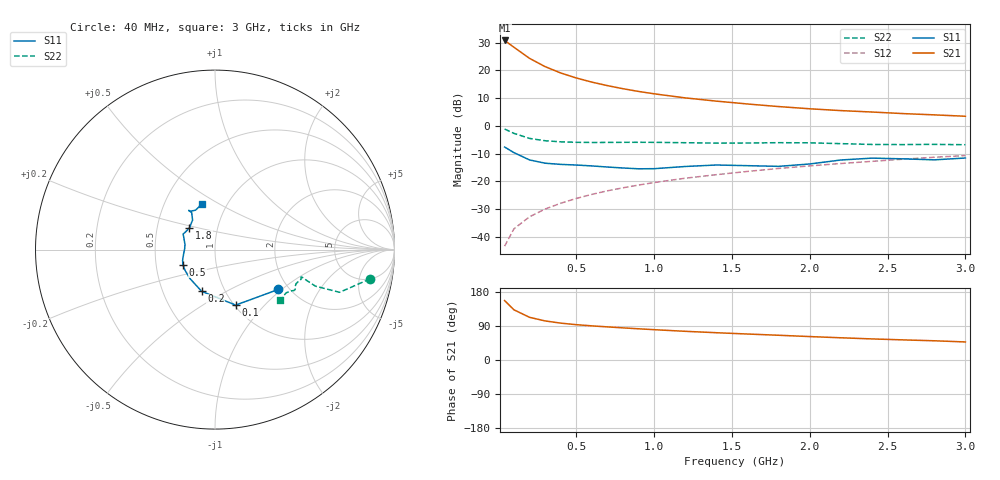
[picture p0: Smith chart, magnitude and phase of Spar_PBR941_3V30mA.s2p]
! Filename:  PBR941H.S2P  Version:  3.0
! NXP part #:  PBR941  Date: July 1998
! Bias condition:  Vce=3V, Ic=30mA
#  MHz  S  MA  R 50
! Freq  S11  S21  S12  S22
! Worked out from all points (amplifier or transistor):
!   21 points, 40 MHz to 3 GHz, reference 50 ohm
!   highest |S21| = 30.8 dB at 40 MHz (marker M1)
!   |S21| within 3 dB of that: start of sweep to 114 MHz
!   unconditionally stable (mu >= 1): 306.6 MHz to 2.554 GHz
!   at 300 MHz: K = 1.00, MSG = 25.6 dB, |S12| = -29.9 dB
!   at 1 GHz: K = 1.10, MAG = 14.1 dB, |S12| = -20.4 dB
!   at 3 GHz: K = 0.99, MSG = 7.1 dB, |S12| = -10.7 dB
!   S11 on the Smith chart (normalised r, x): 40 MHz: 1.76, -0.95; 100 MHz: 1.01, -0.70; 200 MHz: 0.78, -0.38; 500 MHz: 0.69, -0.12; 1.8 GHz: 0.73, +0.18; 3 GHz: 0.77, +0.42
40  0.4167 -32.2  34.49 156.9  0.006845 77.8  0.8788 -10.7
100  0.33 -69.6  26.04 132.4  0.01406 73.2  0.734 -18.9
200  0.244 -107.8  16.44 112.6  0.02313 72.5  0.5951 -20.0
300  0.2131 -131.2  11.67 103.1  0.03187 75.3  0.5406 -18.6
400  0.2029 -145.5  8.971 97.3  0.04049 77.4  0.5168 -17.8
500  0.1976 -155.0  7.289 93.2  0.04941 78.7  0.5065 -17.6
600  0.1903 -161.5  6.14 90.1  0.05851 79.7  0.5032 -17.7
700  0.182 -167.3  5.307 87.4  0.0678 80.7  0.504 -18.0
800  0.1747 -174.0  4.671 84.8  0.07682 80.9  0.5061 -18.4
900  0.169 178.2  4.172 82.4  0.0861 81.0  0.5068 -18.8
1000  0.1698 170.2  3.782 80.0  0.09553 81.0  0.5058 -19.3
1200  0.1859 159.2  3.192 75.7  0.1144 80.7  0.4981 -20.6
1400  0.1978 154.0  2.791 72.0  0.1324 80.3  0.49 -22.8
1600  0.1924 150.1  2.48 68.6  0.1515 80.1  0.4919 -24.9
1800  0.187 139.8  2.228 65.3  0.1714 79.6  0.4989 -26.4
2000  0.2065 127.2  2.032 61.8  0.1906 78.7  0.4956 -27.4
2200  0.2434 122.3  1.885 58.6  0.2104 77.7  0.4793 -28.7
2400  0.2629 123.8  1.777 55.6  0.2301 77.0  0.4635 -31.4
2600  0.2553 123.4  1.665 53.1  0.2517 76.3  0.461 -34.7
2800  0.245 116.3  1.58 50.7  0.2728 75.2  0.465 -36.9
3000  0.2642 105.8  1.491 47.6  0.2922 73.8  0.4584 -37.7
